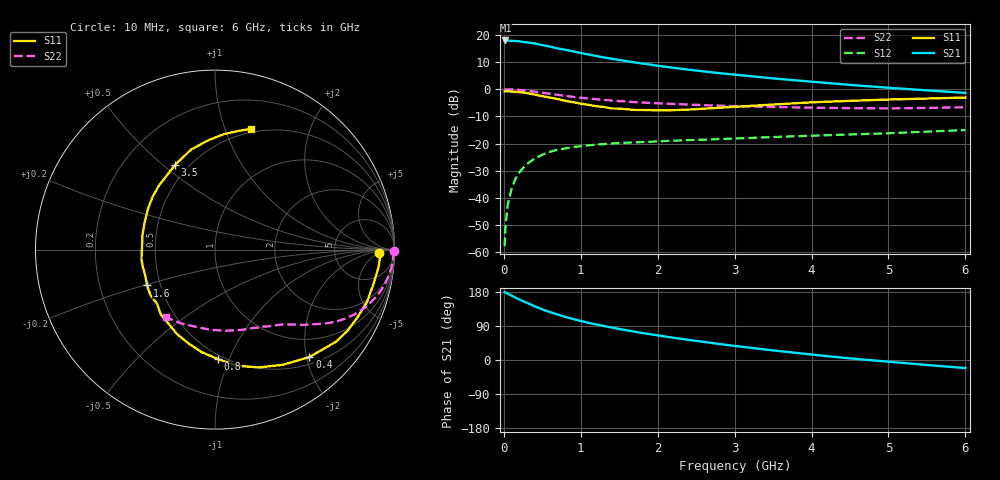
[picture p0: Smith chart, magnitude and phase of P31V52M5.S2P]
! SIEMENS Small Signal Semiconductors
! BFP181
! Si NPN RF Bipolar Junction Transistor in SOT143
! VCE = 1.5 V  IC = 2.5 mA
! Common Emitter S-Parameters:  March  1996
# GHz  S  MA  R  50
!  f  S11  S21  S12  S22
! GHz  MAG  ANG  MAG  ANG  MAG  ANG  MAG  ANG
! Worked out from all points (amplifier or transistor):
!   36 points, 10 MHz to 6 GHz, reference 50 ohm
!   highest |S21| = 17.9 dB at 20 MHz (marker M1)
!   |S21| within 3 dB of that: start of sweep to 713.6 MHz
!   unconditionally stable (mu >= 1): 2.148 GHz to end of sweep
!   at 250 MHz: K = 0.15, MSG = 23.2 dB, |S12| = -28.9 dB
!   at 1.4 GHz: K = 0.74, MSG = 15.6 dB, |S12| = -20.0 dB
!   at 6 GHz: K = 1.14, MAG = 4.6 dB, |S12| = -15.0 dB
!   S11 on the Smith chart (normalised r, x): 10 MHz: 22, -6; 400 MHz: 0.63, -2.05; 800 MHz: 0.47, -0.91; 1.6 GHz: 0.42, -0.21; 3.5 GHz: 0.42, +0.55; 6 GHz: 0.46, +1.23
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0.01  0.9167 -1.3  7.79 179.2  0.0013 92.2  0.9951 -0.6
0.02  0.921 -2.7  7.867 178.5  0.0028 91.4  0.9938 -1.1
0.05  0.9157 -6.4  7.863 175.0  0.0075 87.3  0.9929 -3.0
0.1  0.9028 -12.7  7.706 170.0  0.0147 80.7  0.9887 -5.7
0.2  0.8793 -25.3  7.616 159.9  0.0293 75.1  0.9671 -11.2
0.3  0.8479 -37.2  7.261 151.1  0.0419 68.3  0.9373 -16.2
0.4  0.7969 -48.7  6.931 141.6  0.0531 62.3  0.8997 -20.8
0.5  0.7449 -59.5  6.46 133.5  0.0623 56.8  0.8603 -24.6
0.6  0.7004 -69.6  6.072 126.5  0.0707 52.0  0.8233 -27.8
0.7  0.6592 -79.2  5.613 120.0  0.0769 47.8  0.7868 -30.6
0.8  0.611 -88.3  5.301 113.7  0.0817 44.3  0.7538 -32.9
0.9  0.5765 -97.3  4.965 108.2  0.086 41.3  0.7221 -34.9
1.1  0.5158 -114.3  4.358 98.1  0.0927 36.5  0.6727 -38.3
1.3  0.4715 -129.7  3.834 89.9  0.098 32.7  0.636 -41.2
1.6  0.4279 -152.2  3.27 78.3  0.1041 29.1  0.5932 -44.7
1.8  0.4135 -166.6  2.964 71.2  0.1067 27.7  0.5684 -47.1
2.2  0.412 168.9  2.476 58.8  0.1128 24.8  0.5354 -52.2
2.8  0.4554 139.8  1.973 42.3  0.121 22.0  0.4985 -60.6
3.5  0.5219 115.2  1.58 25.3  0.1319 19.6  0.4705 -72.1
4.5  0.6104 93.5  1.199 4.2  0.1471 15.6  0.4481 -92.6
5.5  0.6731 79.0  0.95 -13.1  0.1659 12.6  0.4524 -114.8
6  0.7022 73.4  0.855 -21.3  0.1773 9.9  0.4661 -126.1
